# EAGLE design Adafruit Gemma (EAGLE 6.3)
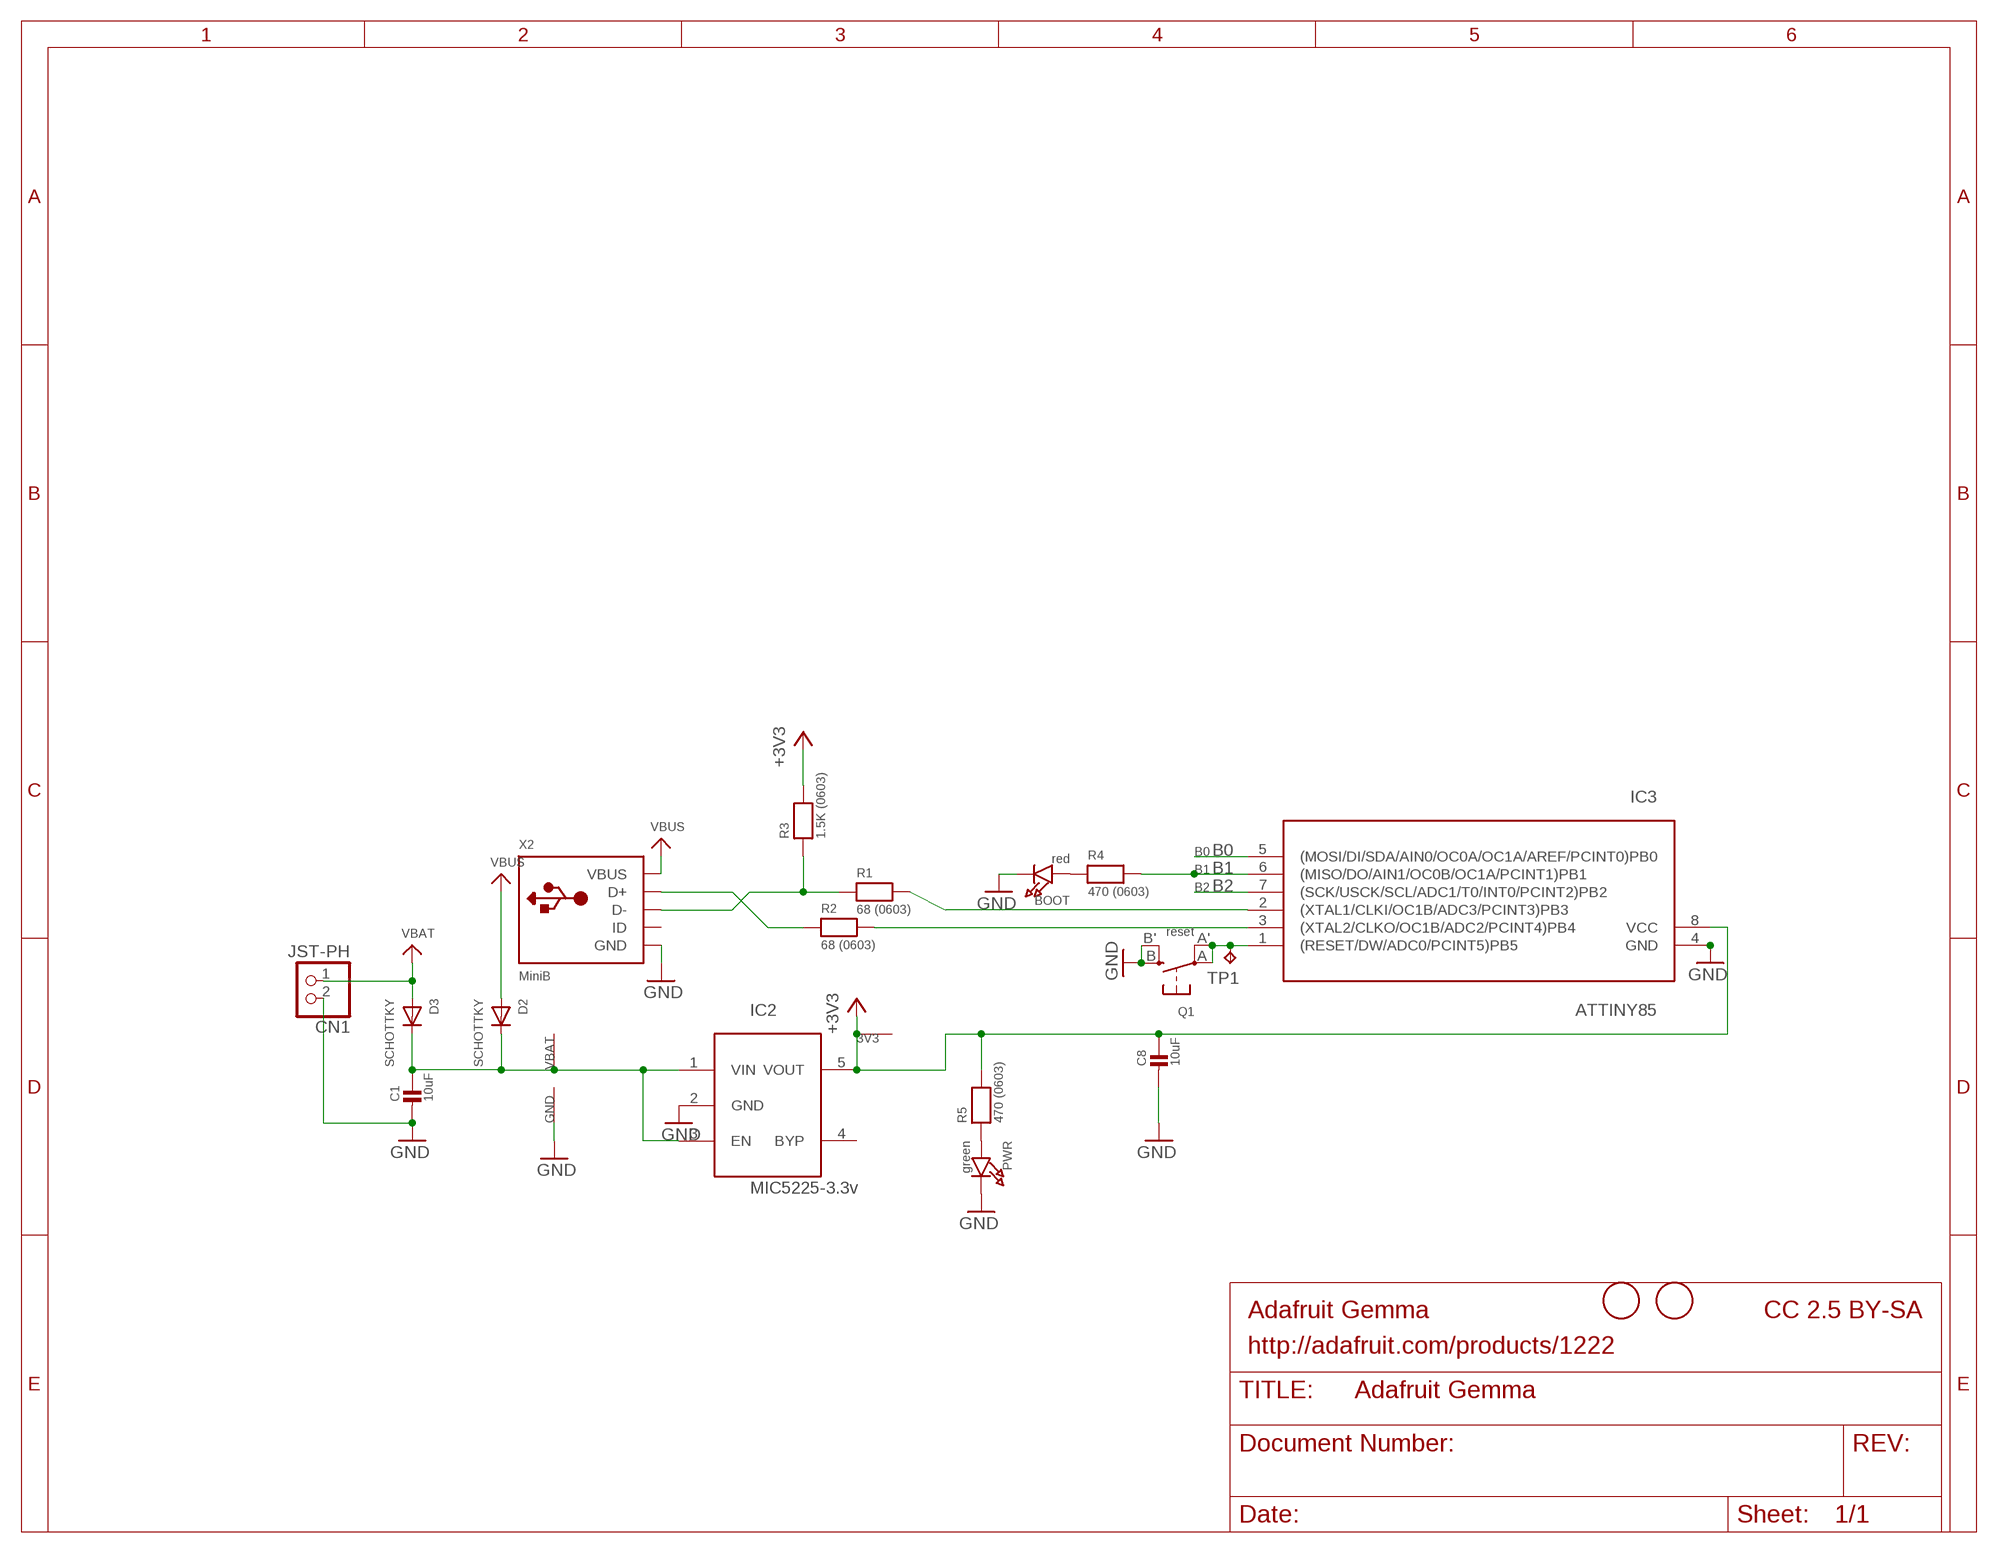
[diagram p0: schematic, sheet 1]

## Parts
3V3  SEWTAP-2.0IN  [SEWINGTAP_2.0]
B0  SEWTAP-2.0IN  [SEWINGTAP_2.0]
B1  SEWTAP-2.0IN  [SEWINGTAP_2.0]
B2  SEWTAP-2.0IN  [SEWINGTAP_2.0]
BOOT  red  LED0805_NOOUTLINE  [CHIPLED_0805_NOOUTLINE]
C1  10uF  CAP_CERAMIC0805-NOOUTLINE  [0805-NO]
C8  10uF  CAP_CERAMIC0805-NOOUTLINE  [0805-NO]
CN1  JST-PH  JST_2PIN-SMT-RA  [JST-PH-2-SMT-RA]
D2  SCHOTTKY  DIODE_SOD-123FL  [SOD-123FL]
D3  SCHOTTKY  DIODE_SOD-123FL  [SOD-123FL]
GND  SEWTAP-2.0IN  [SEWINGTAP_2.0]
IC2  MIC5225-3.3v  LP298XS  [SOT23-5L]
IC3  ATTINY85  ATTINY85V-10S  [SOIC8]
PWR  green  LED0805_NOOUTLINE  [CHIPLED_0805_NOOUTLINE]
Q1  reset  SWITCH_TACT_SMT4.6X2.8  [BTN_KMR2_4.6X2.8]
R1  68 (0603)  RESISTOR_0603_NOOUT  [0603-NO]
R2  68 (0603)  RESISTOR_0603_NOOUT  [0603-NO]
R3  1.5K (0603)  RESISTOR_0603_NOOUT  [0603-NO]
R4  470 (0603)  RESISTOR_0603_NOOUT  [0603-NO]
R5  470 (0603)  RESISTOR_0603_NOOUT  [0603-NO]
TP1  TPB2,54  [B2,54]
U$1  FIDUCIAL  [FIDUCIAL_1MM]
U$6  FIDUCIAL  [FIDUCIAL_1MM]
VBAT  SEWTAP-2.0IN  [SEWINGTAP_2.0]
X2  MiniB  USB_MEDIUM  [USB-MINI_MEDIUM]

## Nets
+3V3: 3V3.P$1(SEW) C8.1 IC2.5(VOUT) IC3.8(VCC) R3.2 R5.2
B0: B0.P$1(SEW) IC3.5((MOSI/DI/SDA/AIN0/OC0A/OC1A/AREF/PCINT0)PB0)
B1: B1.P$1(SEW) IC3.6((MISO/DO/AIN1/OC0B/OC1A/PCINT1)PB1) R4.2
B2: B2.P$1(SEW) IC3.7((SCK/USCK/SCL/ADC1/T0/INT0/PCINT2)PB2)
GND: BOOT.C C1.2 C8.2 CN1.2 GND.P$1(SEW) IC2.2(GND) IC3.4(GND) PWR.C Q1.B'(S1) Q1.B(S) X2.GND X2.GND1(GND) X2.GND2(GND) X2.GND3(GND) X2.GND4(GND)
N$1: IC3.1((RESET/DW/ADC0/PCINT5)PB5) Q1.A'(P1) Q1.A(P) TP1.TP
N$2: R2.1 X2.D+
N$3: IC3.2((XTAL1/CLKI/OC1B/ADC3/PCINT3)PB3) R1.2
N$4: IC3.3((XTAL2/CLKO/OC1B/ADC2/PCINT4)PB4) R2.2
N$5: R1.1 R3.1 X2.D-
N$6: BOOT.A R4.1
N$7: C1.1 D2.C D3.C IC2.1(VIN) IC2.3(EN) VBAT.P$1(SEW)
N$8: PWR.A R5.1
VBAT: CN1.1 D3.A
VBUS: D2.A X2.VBUS
Unconnected: IC2.4(BYP) X2.ID

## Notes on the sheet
- Adafruit Gemma | CC 2.5 BY-SA
- http://adafruit.com/products/1222

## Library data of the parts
3V3 B0 B1 B2 GND VBAT = adafruit:SEWTAP
BOOT PWR = microbuilder:LED: LED
C1 C8 = microbuilder:CAP_CERAMIC: Ceramic Capacitors
CN1 = adafruit:JST_2PIN: JST 2-Pin Connectors of various flavors
D2 D3 = adafruit:DIODE: Diode
IC2 = adafruit:LP298X
IC3 = avr:ATTINY85: MICROCONTROLLER 8 Kbytes FLASH 512 bytes EEPROM 512 bytes RAM 4-channel 10 bit ADC USI
Q1 = microbuilder:SWITCH_TACT_SMT: SMT Tact Switches 6x6mm - Digikey: P12940SCT-ND KMR2 (4.6x2.8mm) - Digikey: 401-1426-1-ND EVQ-PQHB55 - Light Touch, 160GF (4.5x4.5mm) - Digikey: P8090SCT-ND KMT0 - KMT021 NGJ LHS (etc.) IP68/Waterproof - Digikey: CKN10289CT-ND
R1-R5 = microbuilder:RESISTOR: Resistors
TP1 = testpad:TP: Test pad
U$1 U$6 = adafruit:FIDUCIAL: For use by pick and place machines to calibrate the vision/machine, 1mm
X2 = microbuilder:USB: USB Connectors USBMINIB - Surface Mount Female Mini-B USB Connector 4UConnector: 06564

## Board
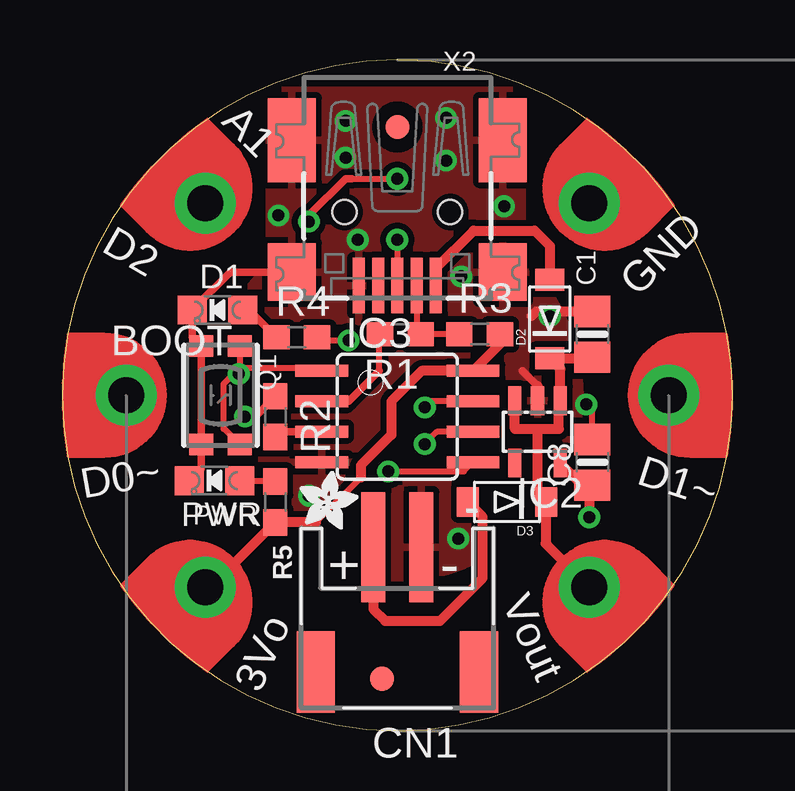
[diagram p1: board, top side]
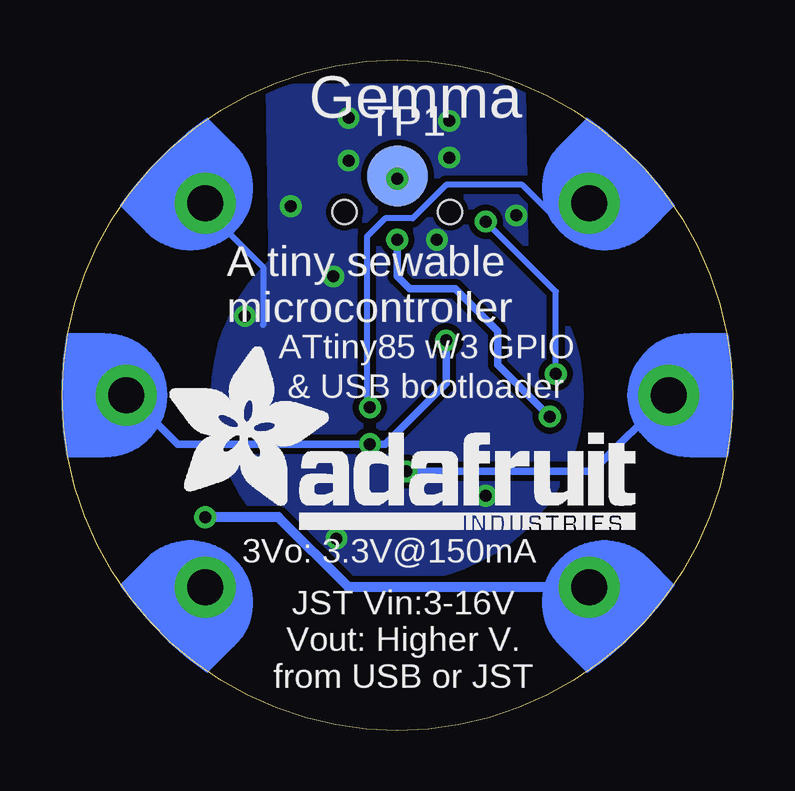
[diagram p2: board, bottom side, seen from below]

Size 27.94 x 27.94 mm. Coordinates in mm from the lower left corner, seen from the top.
Outline: 0,13.97 arc90 13.97,0 arc90 27.94,13.97 arc90 13.97,27.94 arc90 0,13.97
Copper layers (1*16): Top 0.035mm / dielectric 1.5mm / Bottom 0.035mm
Design rules "adafruit *": minimum track width 8mil, minimum drill 15.5mil, track to track 10mil, track to pad 10mil, pad to pad 12mil, via to via 10mil, smd to smd 8mil, copper to edge 10mil, drill to drill 8mil, minimum pad ring 10mil, minimum via ring 8mil, stop-mask expansion 4mil, vias tented up to drill 20mil, thermal gap 10mil

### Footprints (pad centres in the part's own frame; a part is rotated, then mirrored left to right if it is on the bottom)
SEWINGTAP_2.0 = drill 1.5 pad 2.54: P$1 0,0
CHIPLED_0805_NOOUTLINE = smd 1.2 x 1.2: A 0,-1.05; C 0,1.05
0805-NO = smd 1.3 x 1.5: 1 -0.95,0; 2 0.95,0
JST-PH-2-SMT-RA = smd 1 x 4.6: 1 1,-3.7; 2 -1,-3.7 | smd 1.6 x 3.4: NC1 -3.4,1.5; NC2 3.4,1.5
SOD-123FL = smd 0.91 x 1.22: A 1.637,0; C -1.637,0
SOT23-5L = smd 0.55 x 1.2: 1 -0.95,-1.3; 2 0,-1.3; 3 0.95,-1.3; 4 0.95,1.3; 5 -0.95,1.3
SOIC8 = smd 0.5 x 2.2: 1 -1.905,-3.154; 2 -0.645,-3.154; 3 0.625,-3.154; 4 1.895,-3.154; 5 1.905,3.154; 6 0.635,3.154; 7 -0.635,3.154; 8 -1.905,3.154
BTN_KMR2_4.6X2.8 = smd 0.9 x 1: A 2.05,0.8; A' -2.05,0.8; B 2.05,-0.8; B' -2.05,-0.8
0603-NO = smd 1.1 x 1: 1 -0.85,0; 2 0.85,0
B2,54 = smd 2.54 x 2.54: TP 0,0
FIDUCIAL_1MM = smd 1 x 1: 1 0,0
USB-MINI_MEDIUM = smd 0.5 x 2.308: D+ 0,4.064; D- -0.8,4.064; GND 1.6,4.064; ID 0.8,4.064; VBUS -1.6,4.064 | smd 2 x 3.5: GND1 -4.4,-2; GND4 4.4,-2 | smd 2 x 2.4: GND2 -4.4,3.5; GND3 4.4,3.5 | hole 1: -2.2,1; 2.2,1

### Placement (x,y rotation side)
3V3  5.97,5.97 135 top
B0  2.67,13.97 90 top
B1  25.27,13.97 270 top
B2  5.97,21.97 45 top
BOOT  6.48,17.53 90 top
C1  22.1,16.51 90 top
C8  22.1,11.18 90 top
CN1  13.97,3.94 180 top
D2  20.32,17.14 90 top
D3  18.54,9.53 180 top
GND  21.97,21.97 315 top
IC2  19.81,12.45 180 top
IC3  13.97,13.08 270 top
PWR  6.35,10.41 90 top
Q1  6.6,13.97 270 top
R1  14.1,16.51 180 top
R2  8.89,13.08 270 top
R3  17.4,16.51 0 top
R4  9.78,16.38 0 top
R5  8.89,9.53 270 top
TP1  13.97,23.11 0 bottom
U$1  13.97,25.15 0 top
U$2  [ADAFRUIT_2.5MM]  9.91,8.38 0 top
U$6  13.34,2.16 0 top
U$7  [ADAFRUIT_TEXT_20MM]  23.62,8.38 0 bottom
VBAT  21.97,5.97 225 top
X2  13.97,22.61 180 top

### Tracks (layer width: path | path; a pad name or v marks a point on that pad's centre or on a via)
+3V3  (via drill 0.5)
  Top 0.254: 3V3.P$1 6.18,5.97 | 12.45,10.54 10.58,8.68
  Top 0.406: IC2.5 21.68,10.23 C8.1 21.97,10.1 v21.97,8.89 | 17.51,14.99 IC3.8 | IC3.8 14.99,14.99 13.72,13.72 13.72,12.32 12.45,11.05 12.45,10.54 | 10.58,8.68 R5.2 6.18,5.97 | R3.2 18.25,16.11 IC3.8
  Bottom 0.406: 3V3.P$1 16,5.97 18.92,8.89 v21.97,8.89
B0  (via drill 0.5)
  Top 0.254: v13.59,10.8 16.74,10.8 IC3.5
  Bottom 0.305: B0.P$1 5.84,10.8 v13.59,10.8
B1  (via drill 0.5)
  Top 0.254: R4.2 10.76,16.26 v11.94,16.26 | IC3.6 15.62,12.45 v15.11,11.94
  Bottom 0.254: 25.27,13.59 B1.P$1
  Bottom 0.305: B1.P$1 25.15,13.97 23.11,11.94 v15.11,11.94 14.48,11.94 11.94,14.48 v11.94,16.26
B2  (via drill 0.5)
  Top 0.254: IC3.7 15.37,13.72 v15.11,13.46
  Bottom 0.254: B2.P$1 5.97,21.59 7.62,21.59 8.76,22.73 11.94,22.73 13.34,21.34 14.48,21.34 15.24,20.57 15.24,13.59 v15.11,13.46
GND  (via drill 0.5)
  Top 0.254: GND.P$1 22.1,21.84 | 10.18,9.67 v10.29,9.78 | C8.2 22.1,13.34 v21.84,13.59 | 19.81,14.22 IC2.2
  Top 0.305: PWR.C 5.8,10.92 Q1.B Q1.B' 5.43,16.4 BOOT.C 7.01,19.11 X2.GND3 | 19.81,14.35 19.18,14.99
  Top 0.406: C1.2 19.75,17.46 19.56,17.27 | IC2.2 19.81,14.35
  Bottom 0.254: 19.56,16.89 19.56,19.3 21.97,21.72 GND.P$1 | v21.84,13.59 21.21,13.59
  other vias: 12.32,20.45 16.51,8 11.81,25.4 16,25.53 16,23.75 18.41,21.84 11.81,23.88 16.64,18.92 9.02,21.46 20.32,17.27
  pour Bottom: 6.35,13.97 arc90 13.97,6.35 arc90 21.59,13.97 arc90 13.97,21.59 arc90
  pour Bottom: 8.76,26.8 8.64,18.92 19.18,18.92 19.3,26.8
  pour Top: 6.35,13.97 arc90 13.97,6.35 arc90 21.59,13.97 arc90 13.97,21.59 arc90
  pour Top: 8.64,26.67 8.64,18.92 19.18,18.92 19.18,26.67
N$1  (via drill 0.5)
  Top 0.254: Q1.A' 7.4,15.11 | 7.4,15.11 7.37,15.11 v7.37,14.86 | 7.4,15.11 6.73,14.44 6.73,12.57 6.75,12.57 Q1.A | 12.07,22.99 v13.97,22.99 | 7.4,15.11 10.69,15.11 IC3.1
  Top 0.305: 12.07,22.99 11.81,22.99 10.29,21.46 v10.29,21.21
  Bottom 0.254: v7.37,14.86 7.37,18.29 v10.29,21.21 | 14.48,22.61 14.35,22.61 v13.97,22.99 TP1.TP
N$2  (via drill 0.5)
  Top 0.254: v13.97,20.45 X2.D+
  Top 0.305: R2.1 8.04,13.08 v7.62,13.08
  Bottom 0.305: v7.62,13.08 9.78,15.24 9.78,16.64 11.56,18.41 13.46,18.41 13.97,18.92 v13.97,20.45
N$3
  Top 0.254: 11.95,13.73 IC3.2 | 13.21,14.99 13.21,16.47 R1.2
  Top 0.305: 11.95,13.73 13.21,14.99
N$4
  Top 0.305: IC3.3 9.12,12.46 R2.2
N$5
  Top 0.254: R3.1 R1.1 14.77,16.69 X2.D-
N$6
  Top 0.305: BOOT.A 7.79,17.53 R4.1
N$7
  Top 0.254: 21.94,15.4 C1.1
  Top 0.406: 19.81,12.57 18.86,12.57 IC2.3 | 19.81,12.57 20.7,12.57 20.7,13.75 IC2.1 20.76,15.07 D2.C 22.05,15.51 C1.1 | 19.81,12.57 19.81,9.85 19.85,9.85 D3.C 20.18,7.8 20.14,7.8 VBAT.P$1
N$8
  Top 0.254: PWR.A 8.85,10.41 R5.1
VBAT
  Top 0.406: CN1.1 12.97,5.06 13.46,4.57 15.75,4.57 17.53,6.35 17.53,8.9 D3.A
VBUS
  Top 0.406: X2.VBUS 15.57,19.25 17.14,20.83 19.69,20.83 20.32,20.19 D2.A

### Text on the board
tPlace: A1 | D2 | D1 | GND | D0~ | D1~ | PWR | + | - | Vout | 3Vo
bPlace: Gemma | A tiny sewable / microcontroller | ATtiny85 w/3 GPIO | & USB bootloader | 3Vo: 3.3V@150mA | JST Vin:3-16V / Vout: Higher V. / from USB or JST
tDocu: SCL/SCK | GND | SDA/MOSI | MISO | 3-16VDC

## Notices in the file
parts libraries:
microbuilder: This work is placed in the public domain, and may be freely used for commercial and non-commercial work with the following conditions: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
